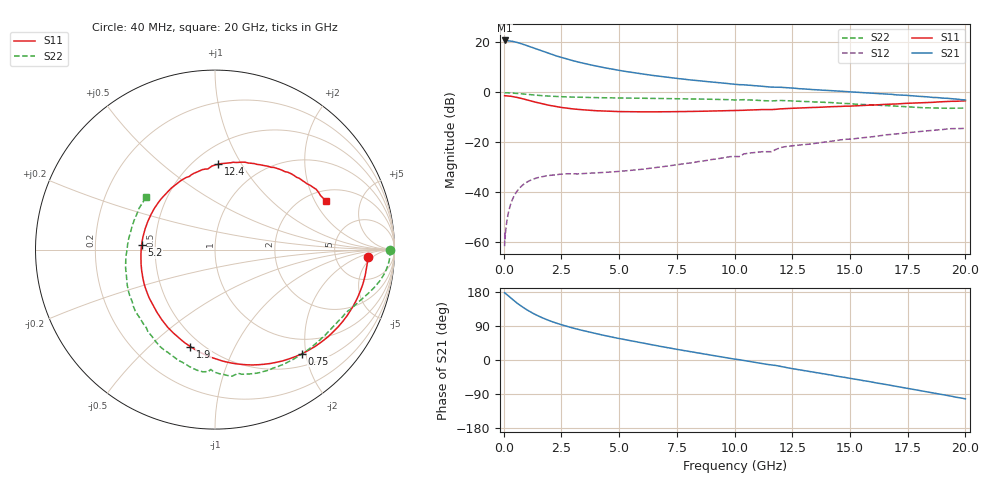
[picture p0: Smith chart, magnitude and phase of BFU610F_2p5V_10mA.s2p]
! Filename:  P:\Prog\Test\Noise\ATS_data\Testdata_Net\SplitFiles\BFU610_2W_A5_HighFreq_2.5V_10mA_D.s2p
! Date/Time: Wed 10/Aug/2011 16:55:36
! BFU610_2W_A5_HighFreq_Bias6_2.5V_1mA_10mA_R.s2p
! MDIF S-parameter v. bias file
! BFU610_2W_A5_HighFreq_2.5V_1mA_10mA
! Date/time Mon Aug 08 14:04:20 2011
! VAR V_out= 2.5010
! VAR I_out= 10.0050
! VAR V_in= 0.9267
! VAR I_in= 0.0950
! Device data file deembeded for feedlines and parallel
! Original file: \SplitFiles\BFU610_2W_A5_HighFreq_2.5V_10mA_R.s2p
! Feed-files: PR003V01_101208_Feed1.s2p, PR003V01_101208_Feed2.s2p
! Parallel-file: PR003V01_101208_Par.s2p
# MHz S MA R 50
!  Freq-MHz  S11-mag  S11-arg  S21-mag  S21-arg  S12-mag  S12-arg  S22-mag  S22-arg
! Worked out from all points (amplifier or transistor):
!   167 points, 40 MHz to 20 GHz, reference 50 ohm
!   highest |S21| = 20.7 dB at 40 MHz (marker M1)
!   |S21| within 3 dB of that: start of sweep to 1.288 GHz
!   unconditionally stable (mu >= 1): 2.26 GHz to end of sweep
!   at 550 MHz: K = 0.26, MSG = 30.0 dB, |S12| = -39.9 dB
!   at 4.2 GHz: K = 1.89, MAG = 15.7 dB, |S12| = -32.1 dB
!   at 20 GHz: K = 1.52, MAG = 1.4 dB, |S12| = -14.4 dB
!   S11 on the Smith chart (normalised r, x): 40 MHz: 12, -3; 750 MHz: 0.71, -1.93; 1.9 GHz: 0.43, -0.68; 5.2 GHz: 0.42, +0.03; 12.4 GHz: 0.65, +0.80; 20 GHz: 2.48, +2.47
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40  0.8524 -2.7  10.86 177.6  0.0008377 81.8  0.9734 -0.2
50  0.8494 -3.3  10.82 177.4  0.001511 70.4  0.9745 -0.4
60  0.8542 -4.1  10.85 176.4  0.001167 73.6  0.9755 -0.6
180  0.8464 -12.7  10.74 170.5  0.003457 82.5  0.974 -2.9
400  0.82 -27.9  10.39 158.9  0.007572 75.1  0.9618 -6.5
550  0.7951 -37.8  10.01 151.6  0.01011 69.5  0.9493 -8.7
750  0.7561 -50.1  9.394 142.6  0.01303 63.0  0.9301 -11.3
950  0.7149 -61.5  8.749 134.5  0.01543 57.3  0.9111 -13.5
1200  0.6665 -74.4  7.958 125.5  0.01772 51.2  0.8882 -15.9
1500  0.6137 -88.2  7.089 116.2  0.01976 45.7  0.8655 -18.4
1900  0.5574 -104.3  6.107 105.7  0.0215 40.4  0.8415 -21.3
2500  0.4973 -124.3  4.969 93.0  0.02302 35.8  0.8128 -25.4
2900  0.4694 -135.5  4.407 86.0  0.02345 33.4  0.8029 -27.9
3400  0.4474 -147.9  3.852 78.2  0.0236 34.0  0.7912 -31.2
4200  0.4229 -165.4  3.207 66.9  0.02483 35.4  0.7785 -36.5
5200  0.4097 176.2  2.643 54.3  0.02662 39.4  0.7668 -43.4
6800  0.4066 151.5  2.071 35.9  0.0321 45.5  0.7506 -54.9
10200  0.4319 109.3  1.419 0.8  0.05174 50.3  0.703 -79.9
12400  0.476 87.7  1.22 -21.7  0.08406 41.8  0.6736 -100.4
13400  0.497 78.2  1.13 -31.7  0.09393 35.5  0.6417 -110.5
16800  0.5794 49.6  0.9104 -67.4  0.1437 11.9  0.5344 -154.6
20000  0.6748 23.7  0.7016 -102.5  0.1905 -20.8  0.4823 142.4
